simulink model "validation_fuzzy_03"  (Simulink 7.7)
settings: Solver=VariableStepDiscrete  StartTime=0.0  StopTime=100  RelTol=1e-3
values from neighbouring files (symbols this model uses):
  A = [0.9944 -0.1203 -0.4302    [process_model02.m]
  B = [1 0    [process_model02.m]
  C = [1 0 0    [process_model02.m]
  D = zeros(2,2)    [process_model02.m]
  Ts = 0.1    [process_model02.m]
  x0 = [0.01 0.02 0.03]    [process_model02.m]
libraries: simulink x6, fuzblock x1

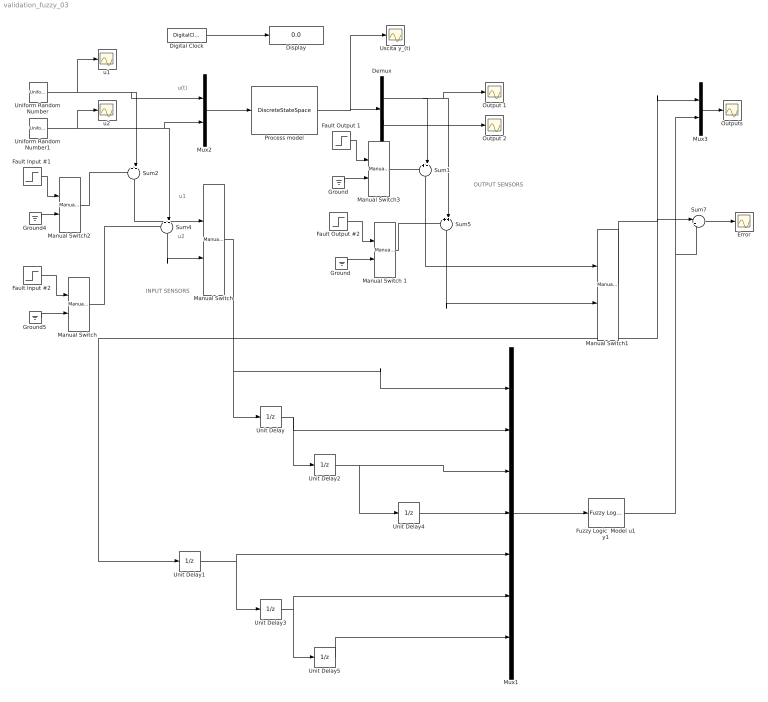
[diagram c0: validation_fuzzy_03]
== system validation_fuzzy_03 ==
  note: u(t)
  note: INPUT SENSORS
  note: OUTPUT SENSORS
  note: u1
  note: u2
  Demux : Demux  Outputs=2
  Digital Clock : DigitalClock  SampleTime=Ts
  Display : Display
  Error : Scope
  Fault Input #1 : Step  Time=50  After=5  SampleTime=Ts
  Fault Input #2 : Step  Time=50  After=5  SampleTime=Ts
  Fault Output #2 : Step  Time=50  After=5  SampleTime=Ts
  Fault Output 1 : Step  Time=50  After=100  SampleTime=Ts
  Fuzzy Logic  Model u1 y1 : fuzblock/Fuzzy Logic  Controller  SystemSampleTime=-1  fis=FM03_u1_y1
  Ground : Ground
  "Ground " : Ground
  Ground4 : Ground
  Ground5 : Ground
  Manual Switch : simulink/Signal Routing/Manual Switch  SystemSampleTime=-1  sw=1  action=0  varsize=off
  "Manual Switch " : simulink/Signal Routing/Manual Switch  SystemSampleTime=-1  sw=0  action=0  varsize=off
  Manual Switch 1 : simulink/Signal Routing/Manual Switch  SystemSampleTime=-1  sw=0  action=0  varsize=off
  Manual Switch1 : simulink/Signal Routing/Manual Switch  SystemSampleTime=-1  sw=1  action=0  varsize=off
  Manual Switch2 : simulink/Signal Routing/Manual Switch  SystemSampleTime=-1  sw=0  action=0  varsize=off
  Manual Switch3 : simulink/Signal Routing/Manual Switch  SystemSampleTime=-1  sw=0  action=0  varsize=off
  Mux1 : Mux  Inputs=7
  Mux2 : Mux  Inputs=2
  Mux3 : Mux  Inputs=2
  Output 1 : Scope
  Output 2 : Scope
  Outputs : Scope
  Process model : DiscreteStateSpace  A=A  B=B  C=C  D=D  X0=x0  SampleTime=Ts
  Sum{1..2,4..5} (4 alike) : Sum  Inputs=++|
  Sum7 : Sum  Inputs=|+-
  Uniform Random Number : UniformRandomNumber  Seed=11  SampleTime=Ts
  Uniform Random Number1 : UniformRandomNumber  Minimum=-0.5  Maximum=0.5  Seed=13  SampleTime=Ts
  Unit Delay{,1..5} (6 alike) : UnitDelay  SampleTime=Ts
  Uscita y_(t) : Scope
  u1 : Scope
  u2 : Scope
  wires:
  Digital Clock/1 -> Display/1
  Mux2/1 -> Process model/1
  Uniform Random Number/1 -> u1/1, Mux2/1, Sum2/2
  Process model/1 -> Uscita y_(t)/1, Demux/1
  Uniform Random Number1/1 -> u2/1, Mux2/2, Sum4/2
  Demux/1 -> Output 1/1, Sum5/2, Sum1/2
  Demux/2 -> Output 2/1
  Sum2/1 -> Manual Switch/1
  Sum4/1 -> Manual Switch/2
  Manual Switch/1 -> Unit Delay/1, Mux1/1
  Unit Delay/1 -> Unit Delay2/1, Mux1/2
  Sum1/1 -> Manual Switch1/1
  Sum5/1 -> Manual Switch1/2
  Unit Delay1/1 -> Unit Delay3/1, Mux1/5
  Manual Switch1/1 -> Unit Delay1/1, Sum7/1, Mux3/1
  Sum7/1 -> Error/1
  Unit Delay2/1 -> Unit Delay4/1, Mux1/3
  Unit Delay3/1 -> Unit Delay5/1, Mux1/6
  Unit Delay4/1 -> Mux1/4
  Unit Delay5/1 -> Mux1/7
  Mux3/1 -> Outputs/1
  Fuzzy Logic  Model u1 y1/1 -> Mux3/2, Sum7/2
  Mux1/1 -> Fuzzy Logic  Model u1 y1/1
  Ground4/1 -> Manual Switch2/2
  Fault Input #1/1 -> Manual Switch2/1
  Fault Input #2/1 -> "Manual Switch "/1
  "Manual Switch "/1 -> Sum4/1
  Manual Switch2/1 -> Sum2/1
  Ground5/1 -> "Manual Switch "/2
  Ground/1 -> Manual Switch3/2
  Fault Output 1/1 -> Manual Switch3/1
  "Ground "/1 -> Manual Switch 1/2
  Fault Output #2/1 -> Manual Switch 1/1
  Manual Switch 1/1 -> Sum5/1
  Manual Switch3/1 -> Sum1/1
